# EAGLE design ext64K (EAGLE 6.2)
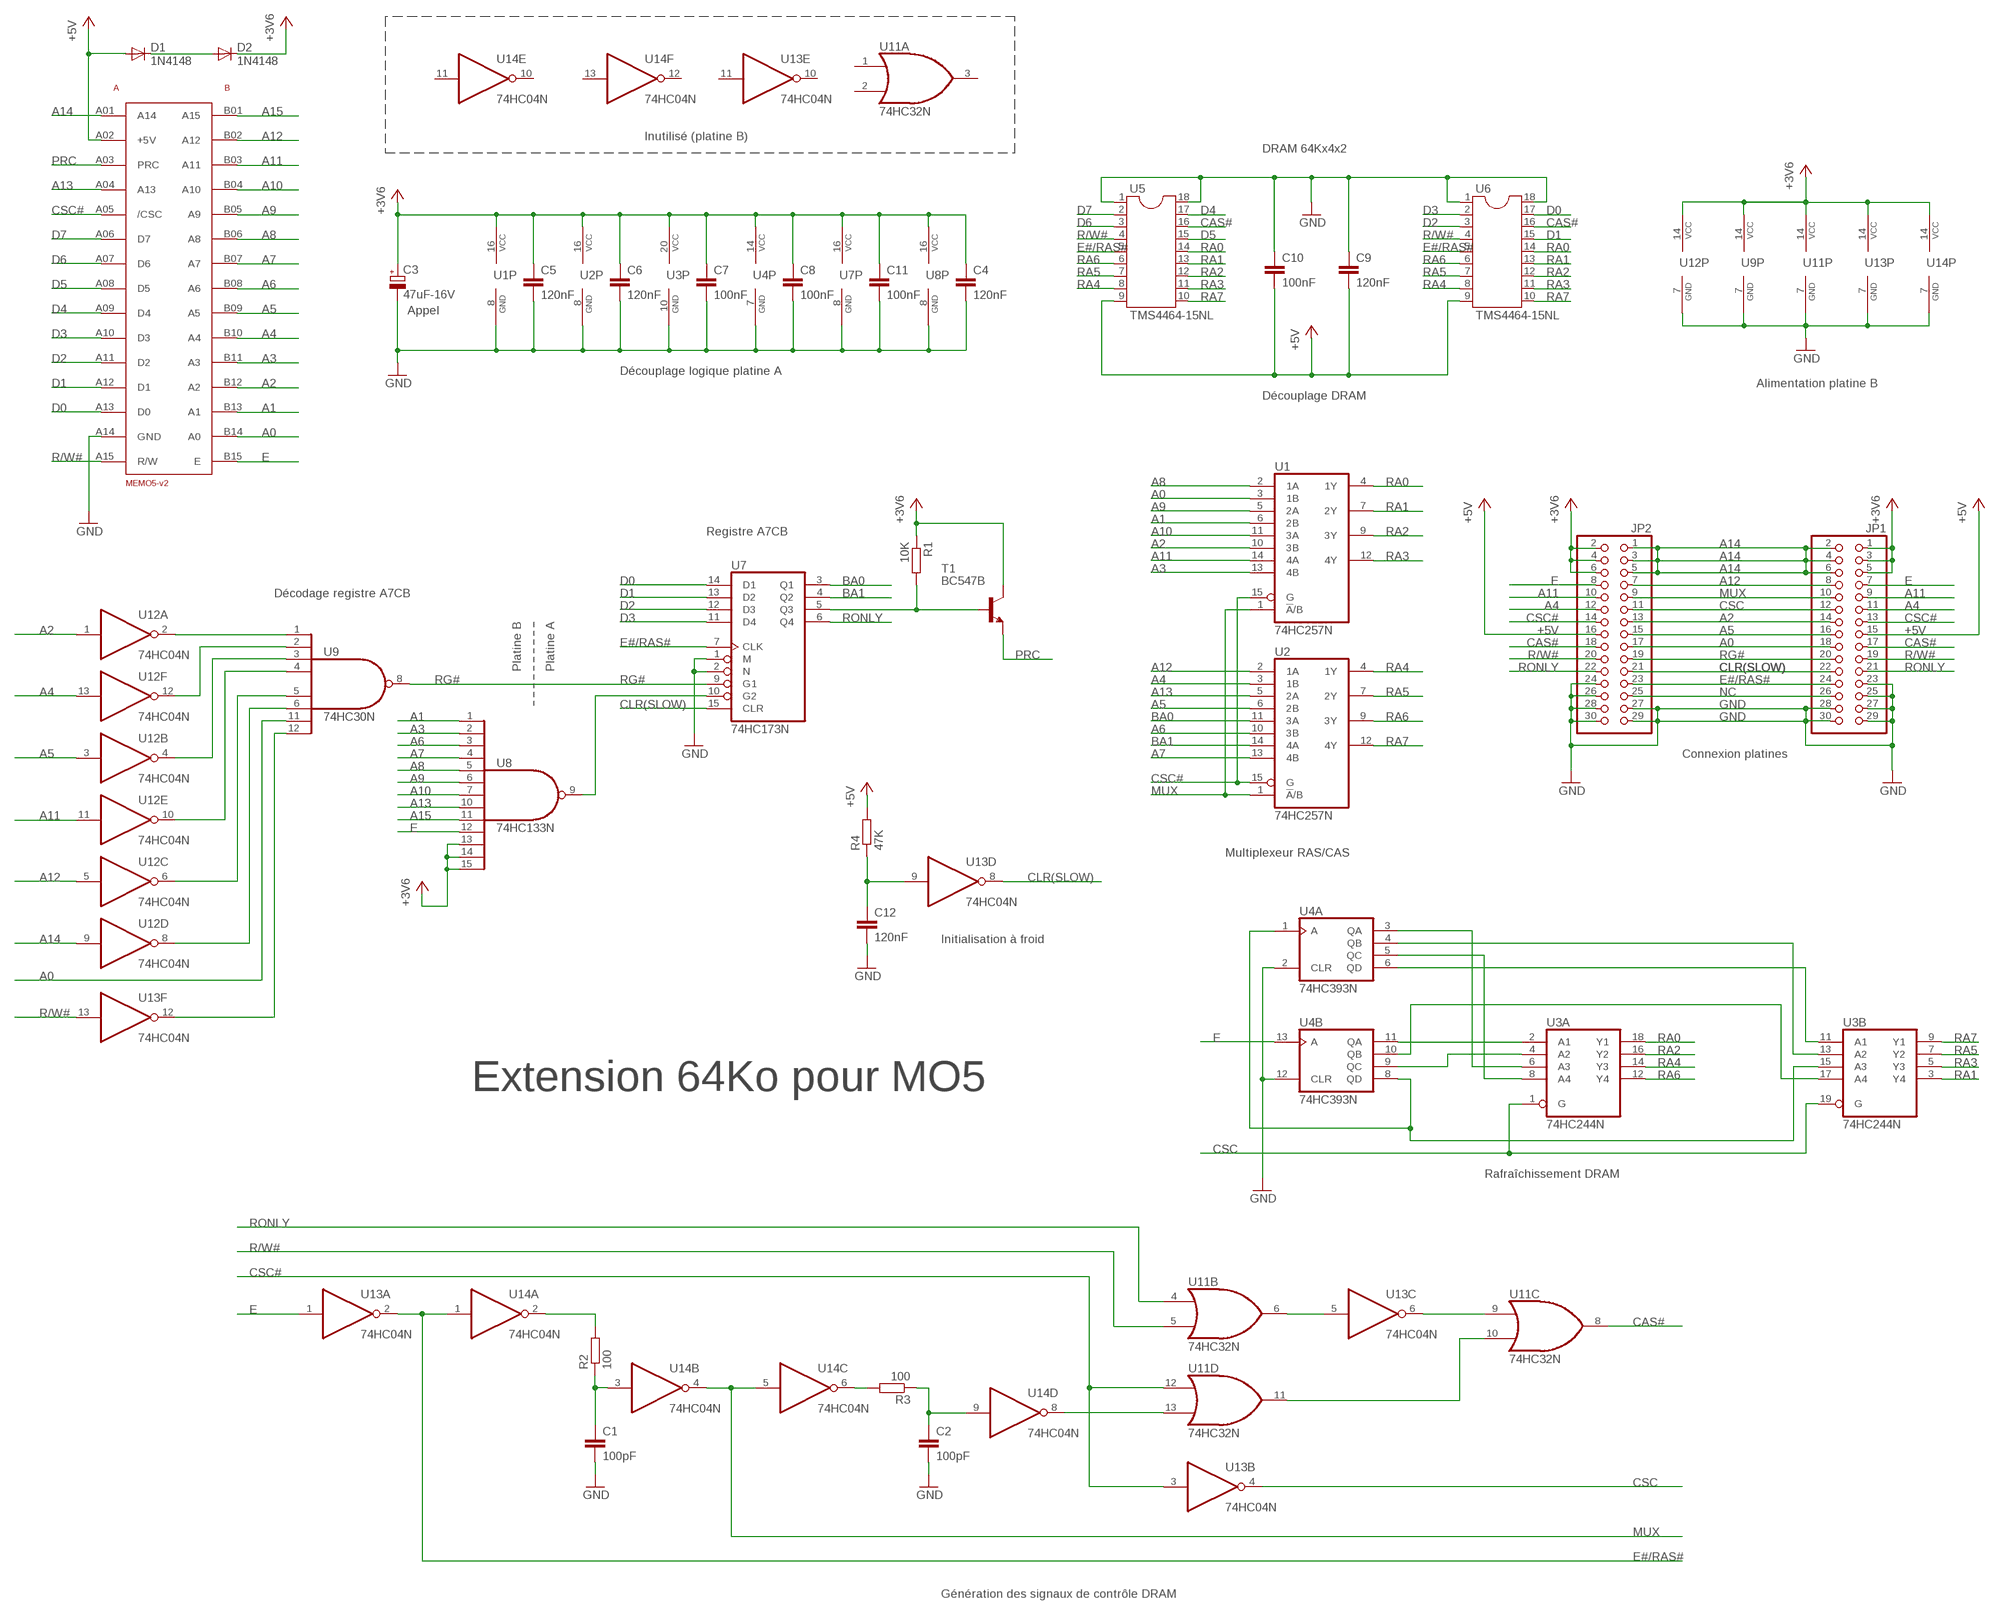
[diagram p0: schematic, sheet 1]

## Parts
BUSMO5  MEMO5-V2ST  [MEMO5]
C1  100pF  C-EU050-025X075  [C050-025X075]
C2  100pF  C-EU050-025X075  [C050-025X075]
C3  47uF-16V  CPOL-EUE5-6  [E5-6]
C4  120nF  C-EU050-024X044  [C050-024X044]
C5  120nF  C-EU050-024X044  [C050-024X044]
C6  120nF  C-EU050-024X044  [C050-024X044]
C7  100nF  C-EU050-024X044  [C050-024X044]
C8  100nF  C-EU050-024X044  [C050-024X044]
C9  120nF  C-EU050-024X044  [C050-024X044]
C10  100nF  C-EU050-024X044  [C050-024X044]
C11  100nF  C-EU050-024X044  [C050-024X044]
C12  120nF  C-EU050-024X044  [C050-024X044]
D1  1N4148  DIODE-DO15-12  [DO15-12]
D2  1N4148  DIODE-DO15-12  [DO15-12]
JP1  PINHD-2X15  [2X15]
JP2  PINHD-2X15  [2X15]
R1  10K  R-EU_0309/12  [0309/12]
R2  100  R-EU_0309/12  [0309/12]
R3  100  R-EU_0309/12  [0309/12]
R4  47K  R-EU_0309/12  [0309/12]
T1  BC547B  [TO92]
U1  74HC257N  74LS257N  [DIL16]
U2  74HC257N  74LS257N  [DIL16]
U3  74HC244N  74LS244N  [DIL20]
U4  74HC393N  74LS393N  [DIL14]
U5  TMS4464-15NL  DIL18  [DIL18]
U6  TMS4464-15NL  DIL18  [DIL18]
U7  74HC173N  74LS173N  [DIL16]
U8  74HC133N  74S133N  [DIL16]
U9  74HC30N  74ALS30N  [DIL14]
U11  74HC32N  74LS32N  [DIL14]
U12  74HC04N  74ALS04N  [DIL14]
U13  74HC04N  74AS04N  [DIL14]
U14  74HC04N  74AS04N  [DIL14]

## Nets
+3V6: C3.+ C4.1 C5.1 C6.1 C7.1 C8.1 C11.1 D2.C JP1.1 JP1.3 JP1.5 JP2.2 JP2.4 JP2.6 R1.1 T1.3(C) U1.16(VCC) U2.16(VCC) U3.20(P:VCC) U4.14(P:VCC) U7.16(VCC) U8.13(I10) U8.14(I11) U8.15(I12) U8.16(VCC) U9.14(VCC) U11.14(P:VCC) U12.14(P:VCC) U13.14(P:VCC) U14.14(P:VCC)
+5V: BUSMO5.A02(+5V) C9.2 C10.2 D1.A JP1.15 JP2.16 R4.2 U5.9 U6.9
A0: BUSMO5.B14(A0) JP1.18 JP2.17 U1.3(1B) U9.11(I6)
A1: BUSMO5.B13(A1) U1.6(2B) U8.1(I0)
A2: BUSMO5.B12(A2) JP1.14 JP2.13 U1.10(3B) U12.1(A:I)
A3: BUSMO5.B11(A3) U1.13(4B) U8.2(I1)
A4: BUSMO5.B10(A4) JP1.11 JP2.12 U2.3(1B) U12.13(F:I)
A5: BUSMO5.B09(A5) JP1.16 JP2.15 U2.6(2B) U12.3(B:I)
A6: BUSMO5.B08(A6) U2.10(3B) U8.3(I2)
A7: BUSMO5.B07(A7) U2.13(4B) U8.4(I3)
A8: BUSMO5.B06(A8) U1.2(1A) U8.5(I4)
A9: BUSMO5.B05(A9) U1.5(2A) U8.6(I5)
A10: BUSMO5.B04(A10) U1.11(3A) U8.7(I6)
A11: BUSMO5.B03(A11) JP1.9 JP2.10 U1.14(4A) U12.11(E:I)
A12: BUSMO5.B02(A12) JP1.8 JP2.7 U2.2(1A) U12.5(C:I)
A13: BUSMO5.A04(A13) U2.5(2A) U8.10(I7)
A14: BUSMO5.A01(A14) JP1.2 JP1.4 JP1.6 JP2.1 JP2.3 JP2.5 U12.9(D:I)
A15: BUSMO5.B01(A15) U8.11(I8)
A#B(SLOW): U11.13(D:I1) U14.8(D:O)
BA0: U2.11(3A) U7.3(Q1)
BA1: U2.14(4A) U7.4(Q2)
CAS#: JP1.17 JP2.18 U5.16 U6.16 U11.8(C:O)
CLR(SLOW): JP1.22 JP2.21 U7.15(CLR) U13.8(D:O)
CSC: JP1.12 JP2.11 U3.1(A:G) U3.19(B:G) U13.4(B:O)
CSC#: BUSMO5.A05(/CSC) JP1.13 JP2.14 U1.15(G) U2.15(G) U11.12(D:I0) U13.3(B:I)
D0: BUSMO5.A13(D0) U6.17 U7.14(D1)
D1: BUSMO5.A12(D1) U6.15 U7.13(D2)
D2: BUSMO5.A11(D2) U6.3 U7.12(D3)
D3: BUSMO5.A10(D3) U6.2 U7.11(D4)
D4: BUSMO5.A09(D4) U5.17
D5: BUSMO5.A08(D5) U5.15
D6: BUSMO5.A07(D6) U5.3
D7: BUSMO5.A06(D7) U5.2
E: BUSMO5.B15(E) JP1.7 JP2.8 U4.13(B:A) U8.12(I9) U13.1(A:I)
E#/RAS#: JP1.24 JP2.23 U5.5 U6.5 U7.7(CLK) U13.2(A:O) U14.1(A:I)
E(SLOW): C1.1 R2.1 U14.3(B:I)
GND: BUSMO5.A14(GND) C1.2 C2.2 C3.- C4.2 C5.2 C6.2 C7.2 C8.2 C9.1 C10.1 C11.2 C12.2 JP1.23 JP1.25 JP1.27 JP1.28 JP1.29 JP1.30 JP2.24 JP2.26 JP2.27 JP2.28 JP2.29 JP2.30 U1.8(GND) U2.8(GND) U3.10(P:GND) U4.2(A:CLR) U4.7(P:GND) U4.12(B:CLR) U5.1 U5.18 U6.1 U6.18 U7.1(M) U7.2(N) U7.8(GND) U8.8(GND) U9.7(GND) U11.7(P:GND) U12.7(P:GND) U13.7(P:GND) U14.7(P:GND)
MUX: JP1.10 JP2.9 U1.1(!A!/B) U2.1(!A!/B) U14.4(B:O) U14.5(C:I)
N$1: U9.2(I1) U12.12(F:O)
N$2: U9.3(I2) U12.4(B:O)
N$3: U9.4(I3) U12.10(E:O)
N$4: U9.5(I4) U12.6(C:O)
N$5: U9.6(I5) U12.8(D:O)
N$6: D1.C D2.A
N$7: U3.2(A:A1) U4.11(B:QA)
N$10: U3.4(A:A2) U4.9(B:QC)
N$11: U3.6(A:A3) U4.3(A:QA)
N$13: U3.8(A:A4) U4.5(A:QC)
N$19: U9.12(I7) U13.12(F:O)
N$20: C12.1 R4.1 U13.9(D:I)
N$21: U3.15(B:A3) U4.1(A:A) U4.8(B:QD)
N$22: U7.10(G2) U8.9(O)
N$23: U3.11(B:A1) U4.6(A:QD)
N$24: U3.13(B:A2) U4.4(A:QB)
N$26: R2.2 U14.2(A:O)
N$27: U3.17(B:A4) U4.10(B:QB)
N$28: R3.2 U14.6(C:O)
N$30: C2.1 R3.1 U14.9(D:I)
N$32: U11.6(B:O) U13.5(C:I)
N$33: U11.9(C:I0) U13.6(C:O)
N$34: U11.10(C:I1) U11.11(D:O)
N$38: R1.2 T1.2(B) U7.5(Q3)
NC: JP1.26 JP2.25
PRC: BUSMO5.A03(PRC) T1.1(E)
R/W#: BUSMO5.A15(R/W) JP1.19 JP2.20 U5.4 U6.4 U11.5(B:I1) U13.13(F:I)
RA0: U1.4(1Y) U3.18(A:Y1) U5.14 U6.14
RA1: U1.7(2Y) U3.3(B:Y4) U5.13 U6.13
RA2: U1.9(3Y) U3.16(A:Y2) U5.12 U6.12
RA3: U1.12(4Y) U3.5(B:Y3) U5.11 U6.11
RA4: U2.4(1Y) U3.14(A:Y3) U5.8 U6.8
RA5: U2.7(2Y) U3.7(B:Y2) U5.7 U6.7
RA6: U2.9(3Y) U3.12(A:Y4) U5.6 U6.6
RA7: U2.12(4Y) U3.9(B:Y1) U5.10 U6.10
RG#: JP1.20 JP2.19 U7.9(G1) U9.8(O)
RONLY: JP1.21 JP2.22 U7.6(Q4) U11.4(B:I0)
S$6: U9.1(I0) U12.2(A:O)
Unconnected: U11.1(A:I0) U11.2(A:I1) U11.3(A:O) U13.10(E:O) U13.11(E:I) U14.10(E:O) U14.11(E:I) U14.12(F:O) U14.13(F:I)

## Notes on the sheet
- Inutilisé (platine B)
- DRAM 64Kx4x2
- Appel
- Découplage logique platine A
- Alimentation platine B
- Découplage DRAM
- Registre A7CB
- Décodage registre A7CB
- Platine B | Platine A
- Connexion platines
- Multiplexeur RAS/CAS
- Initialisation à froid
- Extension 64Ko pour MO5
- Rafraîchissement DRAM
- Génération des signaux de contrôle DRAM

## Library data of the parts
BUSMO5 = thomson:MEMO5-V2
C1 C2 C4-C12 = rcl:C-EU: CAPACITOR, European symbol
C3 = rcl:CPOL-EU: POLARIZED CAPACITOR, European symbol
D1 D2 = diode:DIODE-: DIODE
JP1 JP2 = pinhead:PINHD-2X15: PIN HEADER
R1-R4 = rcl:R-EU_: RESISTOR, European symbol
T1 = transistor-npn:BC547*: NPN Transistor
U1 U2 = 74xx-us:74*257: Quadruple 2-to 1 line data SELECTOR/MULTIPLEXER
U3 = 74xx-us:74*244: Octal BUFFER and LINE DRIVER, 3-state
U4 = 74xx-us:74*393: Dual 4-bit decade and binary COUNTER
U5 U6 = ic-package:DIL18: Dual In Line / Socket
U7 = 74xx-us:74*173: 4-bit D type REGISTER, 3-state
U8 = 74xx-us:74*133: 13-input NAND gate
U9 = 74xx-us:74*30: 8-input NAND gate
U11 = 74xx-us:74*32: Quad 2-input OR gate
U12-U14 = 74xx-us:74*04: Hex INVERTER

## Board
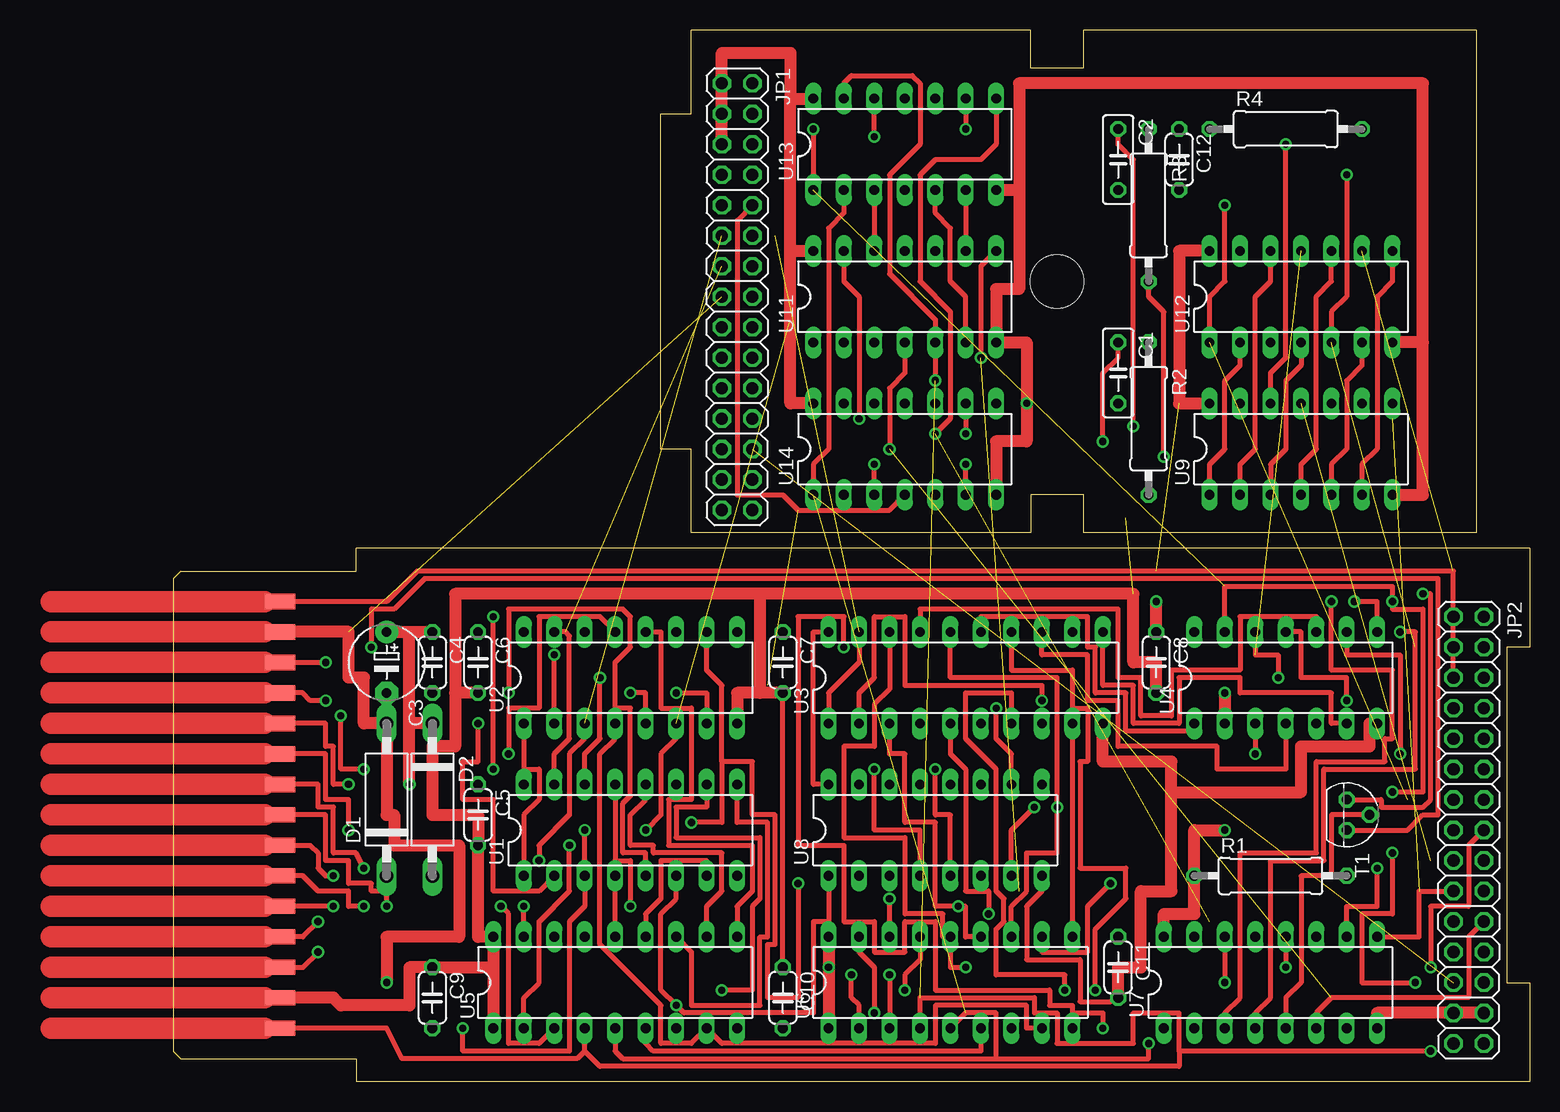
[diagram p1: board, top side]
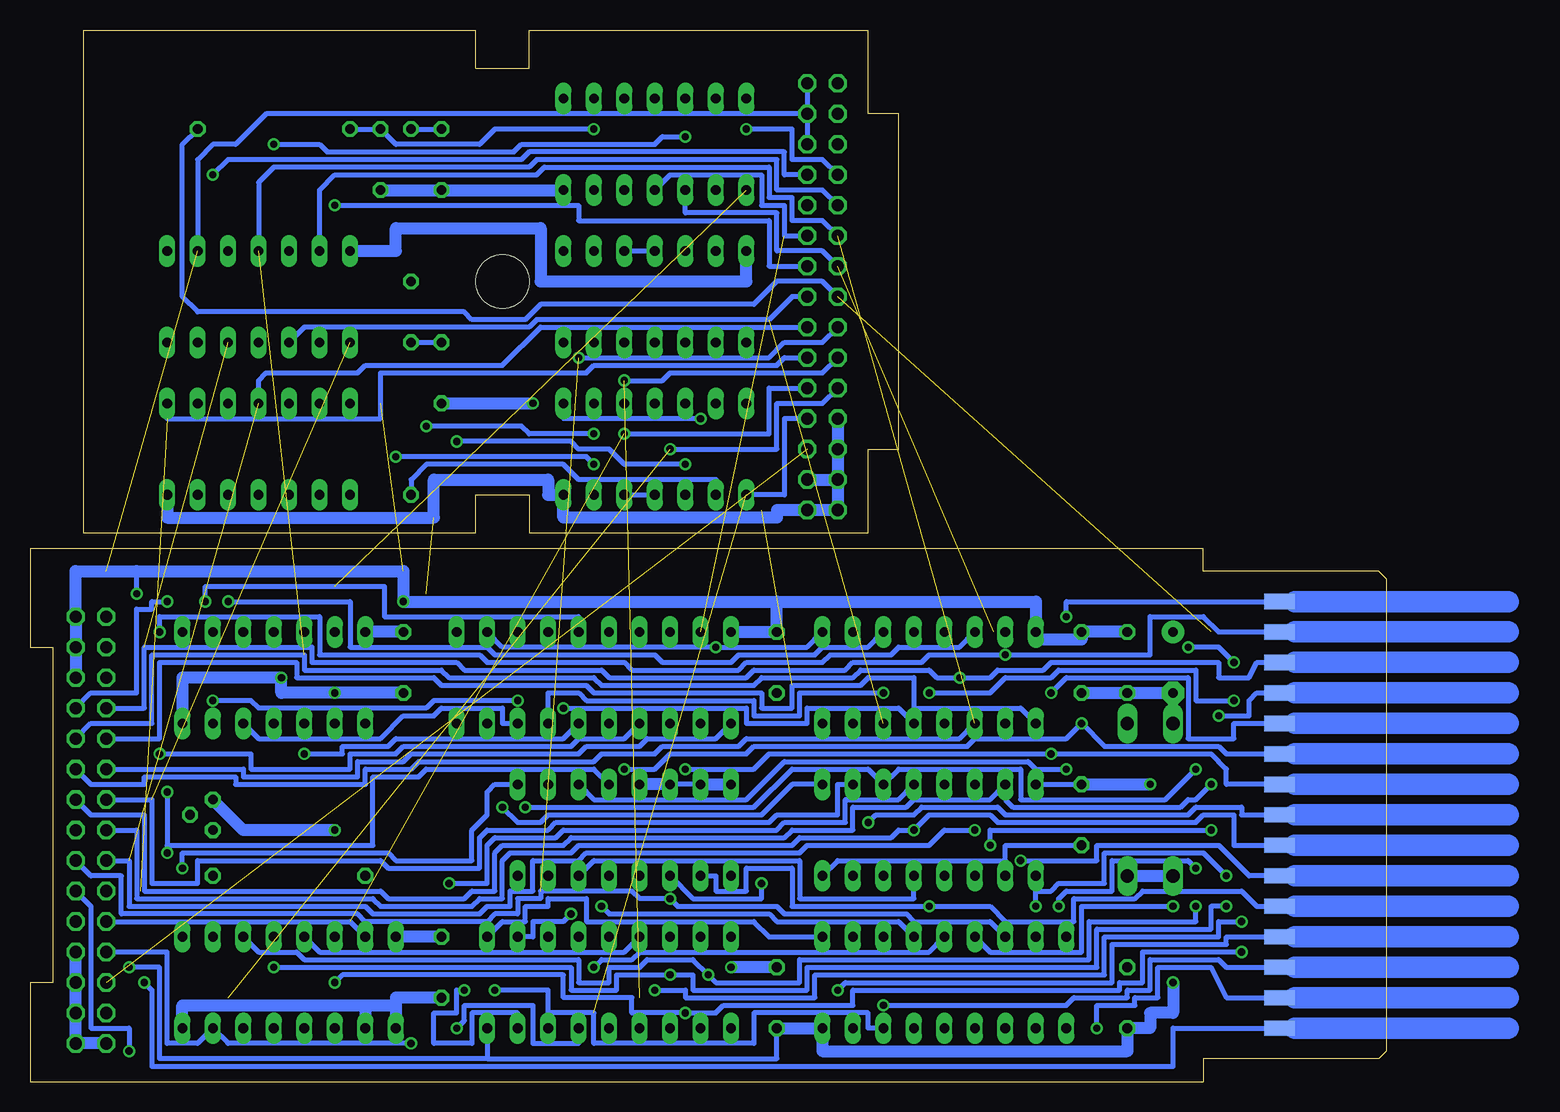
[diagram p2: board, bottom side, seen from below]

Size 113.03 x 87.63 mm. Coordinates in mm from the lower left corner, seen from the top.
Outline: 108.59,87.63 108.59,45.72 75.88,45.72 75.88,48.89 71.44,48.89 71.44,45.72 43.18,45.72 43.18,52.7 40.64,52.7 40.64,80.64 43.18,80.64 43.18,87.63 71.44,87.63 71.44,84.45 75.88,84.45 75.88,87.63 108.59,87.63
Outline: 113.03,44.45 15.24,44.45 15.24,42.54 0.63,42.54 0,41.91 0,2.54 0.63,1.9 15.24,1.9 15.24,0 113.03,0 113.03,8.25 111.12,8.25 111.12,36.2 113.03,36.2 113.03,44.45
Copper layers (1*16): Top 0.035mm / dielectric 1.5mm / Bottom 0.035mm
Design rules: minimum track width 10mil, minimum drill 24mil, track to track 8mil, track to pad 8mil, pad to pad 8mil, via to via 8mil, smd to smd 8mil, copper to edge 40mil, drill to drill 8mil, minimum pad ring 10mil, minimum via ring 8mil, stop-mask expansion 4mil, vias tented up to drill 0mil, thermal gap 10mil
Holes 4.45 mm at 73.66,66.67

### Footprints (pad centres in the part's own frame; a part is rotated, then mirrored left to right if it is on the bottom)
MEMO5 = smd 1.27 x 2.54: A01 -17.78,0; A02 -15.24,0; A03 -12.7,0; A04 -10.16,0; A05 -7.62,0; A06 -5.08,0; A07 -2.54,0; A08 0,0; A09 2.54,0; A10 5.08,0; A11 7.62,0; A12 10.16,0; A13 12.7,0; A14 15.24,0; A15 17.78,0 | smd 1.27 x 2.54 bottom: B01 -17.78,0; B02 -15.24,0; B03 -12.7,0; B04 -10.16,0; B05 -7.62,0; B06 -5.08,0; B07 -2.54,0; B08 0,0; B09 2.54,0; B10 5.08,0; B11 7.62,0; B12 10.16,0; B13 12.7,0; B14 15.24,0; B15 17.78,0
C050-025X075 = drill 0.813 octagon: 1 -2.54,0; 2 2.54,0
E5-6 = drill 0.813 pad 1.905: + -2.54,0 | drill 0.813 pad 1.905 octagon: - 2.54,0
C050-024X044 = drill 0.813 octagon: 1 -2.54,0; 2 2.54,0
DO15-12 = drill 1.118 long: A 6.35,0; C -6.35,0
2X15 = drill 1.016 octagon: 1 -17.78,-1.27; 2 -17.78,1.27; 3 -15.24,-1.27; 4 -15.24,1.27; 5 -12.7,-1.27; 6 -12.7,1.27; 7 -10.16,-1.27; 8 -10.16,1.27; 9 -7.62,-1.27; 10 -7.62,1.27; 11 -5.08,-1.27; 12 -5.08,1.27; 13 -2.54,-1.27; 14 -2.54,1.27; 15 0,-1.27; 16 0,1.27; 17 2.54,-1.27; 18 2.54,1.27; 19 5.08,-1.27; 20 5.08,1.27; 21 7.62,-1.27; 22 7.62,1.27; 23 10.16,-1.27; 24 10.16,1.27; 25 12.7,-1.27; 26 12.7,1.27; 27 15.24,-1.27; 28 15.24,1.27; 29 17.78,-1.27; 30 17.78,1.27
0309/12 = drill 0.813 octagon: 1 -6.35,0; 2 6.35,0
TO92 = drill 0.813 octagon: 1 1.27,0; 2 0,1.905; 3 -1.27,0
DIL16 = drill 0.813 long: 1 -8.89,-3.81; 2 -6.35,-3.81; 3 -3.81,-3.81; 4 -1.27,-3.81; 5 1.27,-3.81; 6 3.81,-3.81; 7 6.35,-3.81; 8 8.89,-3.81; 9 8.89,3.81; 10 6.35,3.81; 11 3.81,3.81; 12 1.27,3.81; 13 -1.27,3.81; 14 -3.81,3.81; 15 -6.35,3.81; 16 -8.89,3.81
DIL20 = drill 0.813 long: 1 -11.43,-3.81; 2 -8.89,-3.81; 3 -6.35,-3.81; 4 -3.81,-3.81; 5 -1.27,-3.81; 6 1.27,-3.81; 7 3.81,-3.81; 8 6.35,-3.81; 9 8.89,-3.81; 10 11.43,-3.81; 11 11.43,3.81; 12 8.89,3.81; 13 6.35,3.81; 14 3.81,3.81; 15 1.27,3.81; 16 -1.27,3.81; 17 -3.81,3.81; 18 -6.35,3.81; 19 -8.89,3.81; 20 -11.43,3.81
DIL14 = drill 0.813 long: 1 -7.62,-3.81; 2 -5.08,-3.81; 3 -2.54,-3.81; 4 0,-3.81; 5 2.54,-3.81; 6 5.08,-3.81; 7 7.62,-3.81; 8 7.62,3.81; 9 5.08,3.81; 10 2.54,3.81; 11 0,3.81; 12 -2.54,3.81; 13 -5.08,3.81; 14 -7.62,3.81
DIL18 = drill 0.813 long: 1 -10.16,-3.81; 2 -7.62,-3.81; 3 -5.08,-3.81; 4 -2.54,-3.81; 5 0,-3.81; 6 2.54,-3.81; 7 5.08,-3.81; 8 7.62,-3.81; 9 10.16,-3.81; 10 10.16,3.81; 11 7.62,3.81; 12 5.08,3.81; 13 2.54,3.81; 14 0,3.81; 15 -2.54,3.81; 16 -5.08,3.81; 17 -7.62,3.81; 18 -10.16,3.81

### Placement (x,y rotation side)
BUSMO5  8.89,22.23 270 top
C1  78.74,59.05 270 top
C2  78.74,76.83 270 top
C3  17.78,34.92 270 top
C4  21.59,34.92 270 top
C5  25.4,22.23 270 top
C6  25.4,34.92 270 top
C7  50.8,34.92 270 top
C8  81.92,34.92 270 top
C9  21.59,6.98 270 top
C10  50.8,6.98 270 top
C11  78.74,9.52 270 top
C12  83.82,76.83 270 top
D1  17.78,23.5 90 top
D2  21.59,23.5 270 top
JP1  46.99,65.41 270 top
JP2  107.95,20.96 270 top
R1  91.44,17.14 0 top
R2  81.28,55.24 270 top
R3  81.28,73.02 270 top
R4  92.71,79.38 0 top
T1  97.79,22.23 270 top
U1  38.1,20.96 0 top
U2  38.1,33.66 0 top
U3  66.04,33.66 0 top
U4  92.71,33.66 0 top
U5  36.83,8.25 0 top
U6  64.77,8.25 0 top
U7  91.44,8.25 0 top
U8  63.5,20.96 0 top
U9  93.98,52.7 0 top
U11  60.96,65.41 0 top
U12  93.98,65.41 0 top
U13  60.96,78.11 0 top
U14  60.96,52.7 0 top

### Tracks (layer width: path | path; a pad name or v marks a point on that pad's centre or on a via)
+3V6  (via drill 0.6)  (1 unrouted)
  Top 0.406: T1.3 100.65,23.5 100.65,22.86 104.14,22.86 104.78,23.5 104.78,40.64 v104.14,40.64 | U8.16 53.34,24.77 53.34,37.46 U3.20
  Top 1.016: U12.14 83.82,69.22 83.82,56.52 U9.14 | U14.14 51.43,56.52 51.43,69.22 | 51.43,69.22 U11.14 | 51.43,69.22 51.43,81.91 | 51.43,81.91 U13.14 | JP1.5 JP1.3 JP1.1 45.72,85.72 51.43,85.72 51.43,81.91 | C8.1 v81.92,40 | C3.+ 19.68,37.46 | 19.68,37.46 C4.1 | D2.C 19.68,29.85 | 19.68,29.85 19.68,37.46 | U7.16 82.55,13.97 85.09,13.97 R1.1 85.09,20.96 v87.63,20.96 | v19.68,24.77 19.68,29.85
  Bottom 0.406: v104.14,40.64 104.14,42.54 | U8.15 U8.14 | U1.16 C5.1
  Bottom 1.016: U12.14 82.55,69.22 82.55,71.12 70.48,71.12 70.48,66.67 53.34,66.67 U11.14 | C8.1 U4.14 | JP2.6 JP2.4 JP2.2 109.22,42.54 104.14,42.54 81.92,42.54 v81.92,40 50.8,40 | 50.8,40 29.21,40 U2.16 29.21,36.83 25.4,36.83 C6.1 C4.1 | 50.8,40 C7.1 U3.20 | v87.63,20.96 95.25,20.96 T1.3 | C11.1 U7.16 | U8.15 U8.16 | U8.14 U8.13 | C5.1 v19.68,24.77
+5V  (via drill 0.6)  (1 unrouted)
  Top 0.406: JP2.16 107.95,19.69 107.95,14.61 104.78,14.61 v104.78,9.52
  Top 1.016: BUSMO5.A02 14.61,37.46 14.61,33.66 15.88,33.66 15.88,29.85 D1.A 17.78,22.23 18.41,22.23 18.41,19.69 23.81,19.69 23.81,12.07 17.78,12.07 v17.78,8.25
  Bottom 0.406: v104.78,9.52 102.23,9.52 102.23,1.9 74.93,1.9 | U6.9 74.93,1.9 | 74.93,1.9 50.8,1.9 C10.2 | R4.2 100.33,78.11 100.33,65.41 99.06,64.14 76.84,64.14 76.2,63.5 71.76,63.5 70.48,64.77 52.7,64.77 50.8,66.67 46.99,66.67 JP1.15
  Bottom 1.016: C10.2 U5.9 46.99,2.54 21.59,2.54 C9.2 19.68,4.45 19.68,5.71 17.78,5.71 v17.78,8.25
A0  (via drill 0.6)  (1 unrouted)
  Top 0.406: v34.29,20.96 U1.3 34.29,14.61 33.02,13.34 33.02,2.54 24.13,2.54 v24.13,4.45
  Bottom 0.406: JP2.17 104.78,18.41 104.78,14.61 85.09,14.61 84.45,13.97 75.56,13.97 74.93,14.61 73.03,14.61 73.03,15.88 71.12,15.88 71.12,18.41 67.31,18.41 66.67,19.05 48.89,19.05 48.26,19.69 38.1,19.69 36.83,20.96 v34.29,20.96 | v24.13,4.45 24.13,6.35 20.96,6.35 20.96,6.98 19.05,6.98 19.05,9.52 14.61,9.52 13.34,6.98 BUSMO5.B14 | U9.11 93.98,58.42 93.34,59.05 85.73,59.05 85.09,59.69 73.66,59.69 70.48,62.86 JP1.18
A1  (via drill 0.6)
  Top 0.406: U8.1 54.61,13.34 53.34,13.34 53.34,5.71 42.54,5.71 v41.91,6.35 40.64,7.62 40.64,13.97 41.91,15.24 U1.6
  Bottom 0.406: v41.91,6.35 26.67,6.35 26.04,6.98 21.59,6.98 21.59,7.62 19.68,7.62 19.68,10.16 13.97,10.16 13.34,9.52 BUSMO5.B13
A2  (via drill 0.6)  (1 unrouted)
  Top 0.406: U1.10 44.45,22.86 41.91,22.86 41.91,20.32 48.89,20.32 48.89,15.24 48.26,14.61 48.26,7.62 v45.72,7.62 | U12.1 86.36,65.41 87.63,66.67 v87.63,73.02
  Bottom 0.406: JP2.13 102.87,23.5 102.87,16.51 99.06,16.51 99.06,18.41 83.82,18.41 83.19,17.78 75.56,17.78 75.56,20.32 74.93,20.96 69.85,20.96 69.22,21.59 51.43,21.59 50.8,22.23 45.72,22.23 45.72,24.77 U1.10 | v45.72,7.62 45.09,8.25 22.86,8.25 22.86,11.43 13.34,11.43 13.34,12.07 BUSMO5.B12 | v87.63,73.02 67.31,73.02 67.31,71.75 51.43,71.75 51.43,67.94 JP1.14
A3  (via drill 0.6)
  Top 0.406: U1.13 36.83,18.41 38.1,18.41 v38.1,14.61
  Bottom 0.406: U8.2 55.88,17.14 55.88,15.88 53.34,15.88 53.34,17.78 49.53,17.78 49.53,14.61 v38.1,14.61 33.02,14.61 31.75,13.34 26.04,13.34 26.04,15.24 20.96,15.24 20.32,15.88 12.07,15.88 10.79,14.61 BUSMO5.B11
A4  (via drill 0.6)  (1 unrouted)
  Top 0.406: U2.3 34.29,28.57 33.02,27.3 33.02,22.23 30.48,19.69 v30.48,18.41
  Bottom 0.406: JP2.12 107.95,24.77 103.51,24.77 103.51,25.4 95.89,25.4 95.89,24.77 85.09,24.77 85.09,26.04 81.28,26.04 80.65,26.67 66.04,26.67 65.41,27.3 60.96,27.3 60.32,27.94 53.97,27.94 53.34,28.57 35.56,28.57 U2.3 | v30.48,18.41 24.13,18.41 24.13,19.69 13.97,19.69 11.43,17.14 BUSMO5.B10 | U12.13 88.9,74.3 87.63,75.56 70.8,75.56 70.17,76.2 51.43,76.2 51.43,73.66 49.53,73.66 49.53,71.75 46.99,71.75 JP1.11
A5  (via drill 0.6)  (1 unrouted)
  Top 0.406: U2.6 41.91,28.57 40.64,27.3 40.64,22.23 v39.37,20.96
  Bottom 0.406: JP2.15 104.14,20.96 104.14,15.24 84.45,15.24 83.82,14.61 76.2,14.61 75.56,15.24 73.66,15.24 73.66,18.41 73.03,19.05 67.95,19.05 67.31,19.69 49.53,19.69 48.89,20.32 41.27,20.32 40.64,20.96 v39.37,20.96 38.1,22.23 33.02,22.23 32.38,21.59 15.88,21.59 15.24,22.23 12.7,22.23 12.7,19.69 BUSMO5.B09 | JP1.16 49.53,65.41 51.43,63.5 70.8,63.5 71.44,62.86 90.17,62.86 U12.3
A6  (via drill 0.6)
  Top 0.406: v52.07,16.51 52.07,6.98 49.53,6.98 49.53,11.43 50.16,11.43 50.16,22.23 48.26,22.23 48.26,26.67 45.72,26.67 | 45.72,26.67 45.72,33.02 44.45,34.29 U2.10 | 45.72,26.67 45.72,21.59 v43.18,21.59
  Bottom 0.406: U8.3 57.78,15.24 52.07,15.24 v52.07,16.51 | v43.18,21.59 42.54,22.23 39.37,22.23 38.73,22.86 32.38,22.86 31.75,22.23 16.51,22.23 15.88,22.86 12.07,22.86 12.07,22.23 BUSMO5.B08
A7  (via drill 0.6)
  Top 0.406: U8.4 62.23,20.96 58.42,20.96 v58.42,26.04 | U2.13 35.56,38.73 30.48,38.73 30.48,31.12 27.94,31.12 v27.94,27.3
  Bottom 0.406: v58.42,26.04 52.7,26.04 51.43,27.3 v27.94,27.3 14.61,27.3 13.34,26.04 13.34,24.77 BUSMO5.B07
A8  (via drill 0.6)
  Top 0.406: U8.5 64.77,22.23 63.5,22.23 v63.5,26.04 | U1.2 30.48,15.88 26.67,15.88 26.67,23.5 24.13,23.5 24.13,26.67 25.4,26.67 v25.4,29.85
  Bottom 0.406: v63.5,26.04 60.96,26.04 59.69,27.3 53.34,27.3 52.7,27.94 34.92,27.94 34.29,28.57 26.67,28.57 v25.4,29.85 23.5,27.94 13.97,27.94 13.34,27.3 BUSMO5.B06
A9  (via drill 0.6)
  Top 0.406: U1.5 39.37,19.05 37.46,19.05 37.46,23.18 38.1,23.81 38.1,31.12 36.83,31.12 36.83,34.92 38.1,36.2 38.1,38.73 37.46,39.37 27.94,39.37 v27.94,32.38
  Bottom 0.406: U8.6 66.04,18.41 48.89,18.41 48.89,15.24 39.37,15.24 U1.5 | v27.94,32.38 26.67,33.66 16.51,33.66 16.51,28.57 12.7,28.57 12.7,29.85 BUSMO5.B05
A10  (via drill 0.6)
  Top 0.406: U8.7 69.85,20.96 v71.76,22.86 | v15.88,26.04 13.97,26.04 v13.97,30.48
  Bottom 0.406: v71.76,22.86 52.7,22.86 49.53,26.04 43.18,26.04 U1.11 40.64,26.04 30.48,26.04 30.48,23.5 18.41,23.5 v15.88,26.04 | v13.97,30.48 11.43,30.48 11.43,31.75 10.79,32.38 BUSMO5.B04
A11  (via drill 0.6)  (1 unrouted)
  Top 0.406: U1.14 34.29,27.3 35.56,28.57 v35.56,33.66
  Bottom 0.406: JP2.10 107.95,29.85 102.87,29.85 102.87,35.56 90.17,35.56 90.17,34.29 78.74,34.29 78.11,33.66 66.04,33.66 65.41,33.02 52.7,33.02 52.07,33.66 44.45,33.66 43.81,34.29 38.1,34.29 37.46,33.66 v35.56,33.66 33.02,33.66 32.38,34.29 28.57,34.29 27.94,34.92 13.97,34.92 13.97,33.66 11.43,33.66 10.79,34.92 BUSMO5.B03 | JP1.9 46.99,74.3 50.8,74.3 50.8,76.83 70.8,76.83 71.44,76.2 92.71,76.2 93.98,74.93 U12.11
A12  (via drill 0.6)  (1 unrouted)
  Top 0.406: U2.2 v31.75,35.56 | v97.79,75.56 97.79,65.41 96.52,64.14 U12.5
  Bottom 0.406: JP2.7 103.51,31.12 103.51,36.2 89.54,36.2 89.54,34.92 77.47,34.92 76.84,34.29 65.41,34.29 64.77,33.66 53.34,33.66 52.7,34.29 45.09,34.29 44.45,34.92 38.73,34.92 38.1,35.56 v31.75,35.56 19.68,35.56 19.68,38.73 15.24,38.73 13.97,37.46 BUSMO5.B02 | JP1.8 50.16,75.56 50.16,77.47 71.44,77.47 72.07,76.83 96.52,76.83 v97.79,75.56
A13  (via drill 0.6)
  Top 0.406: U8.10 69.85,27.3 68.58,28.57 v68.58,31.12 | U2.5 39.37,32.38 v38.1,32.38 | v12.7,31.75 11.43,31.75 10.79,32.38 BUSMO5.A04
  Bottom 0.406: v68.58,31.12 53.34,31.12 53.34,29.85 48.26,29.85 48.26,31.12 40.64,31.12 U2.5 | v38.1,32.38 33.02,32.38 31.75,33.66 27.94,33.66 27.3,34.29 15.88,34.29 15.88,31.75 v12.7,31.75
A14  (1 unrouted)
  Top 0.406: JP2.5 JP2.3 JP2.1 106.68,42.54 20.32,42.54 17.78,40 BUSMO5.A01
  Bottom 0.406: JP1.2 JP1.4 | JP1.4 JP1.6 | JP1.4 93.34,80.64 95.89,78.11 97.79,78.11 99.06,76.83 U12.9
A15  (via drill 0.6)
  Top 0.406: v26.67,26.04 v26.67,38.73
  Bottom 0.406: U8.11 66.04,23.5 53.34,23.5 50.16,26.67 29.85,26.67 29.21,26.04 v26.67,26.04 | v26.67,38.73 26.67,40 BUSMO5.B01
A#B(SLOW)  (via drill 0.6)
  Top 0.406: U11.13 55.88,66.67 57.15,65.41 v57.15,55.24
  Bottom 0.406: v57.15,55.24 68.58,55.24 U14.8
BA0  (via drill 0.6)
  Top 0.406: U7.3 87.63,5.71 88.9,6.98 88.9,19.05 95.25,19.05 95.25,26.67 100.97,26.67 100.97,28.57 101.6,28.57 101.6,34.29 96.52,34.29 v96.52,40
  Bottom 0.406: v96.52,40 86.36,40 86.36,36.2 74.93,36.2 74.3,35.56 60.96,35.56 60.32,34.92 54.61,34.92 53.97,35.56 47.62,35.56 46.99,36.2 43.18,36.2 U2.11
BA1  (via drill 0.6)
  Top 0.406: U7.4 90.17,5.71 91.44,6.98 91.44,18.41 95.89,18.41 95.89,26.04 103.51,26.04 103.51,37.46 v102.23,37.46
  Bottom 0.406: v102.23,37.46 102.23,38.73 88.9,38.73 88.9,35.56 75.56,35.56 74.93,34.92 63.5,34.92 62.86,34.29 53.97,34.29 53.34,34.92 46.99,34.92 46.35,35.56 41.27,35.56 40.64,36.2 35.56,36.2 U2.14
CAS#  (via drill 0.6)  (1 unrouted)
  Top 0.406: U6.16 v59.69,15.24 | U11.8 67.31,67.94 v67.31,60.32
  Bottom 0.406: JP2.18 107.95,17.14 105.41,17.14 105.41,13.97 85.73,13.97 85.09,13.34 74.93,13.34 74.3,13.97 72.39,13.97 72.39,15.24 70.48,15.24 70.48,15.88 62.86,15.88 62.23,15.24 v59.69,15.24 59.05,14.61 50.8,14.61 50.16,13.97 40,13.97 39.37,13.34 33.02,13.34 U5.16 | v67.31,60.32 51.43,60.32 50.16,61.59 46.99,61.59 JP1.17
CLR(SLOW)  (via drill 0.6)  (1 unrouted)
  Top 0.406: U13.8 68.58,78.11 67.31,76.83 63.5,76.83 62.23,75.56 62.23,66.67 64.77,64.14 64.77,55.24 v63.5,53.97
  Bottom 0.406: JP2.21 86.36,13.34 U7.15 | v63.5,53.97 51.43,53.97 51.43,57.78 JP1.22
CSC  (1 unrouted)
  Top 0.406: U3.19 57.15,34.92 54.61,32.38 U3.1
  Bottom 0.406: JP2.11 95.25,26.04 95.25,25.4 85.73,25.4 85.73,26.67 81.92,26.67 81.28,27.3 67.31,27.3 66.67,27.94 62.23,27.94 61.59,28.57 55.88,28.57 U3.1 | U13.4 59.69,75.56 52.07,75.56 52.07,73.02 50.16,73.02 50.16,70.48 JP1.12
CSC#  (via drill 0.6)  (1 unrouted)
  Top 0.406: U1.15 31.75,27.3 33.02,28.57 33.02,37.15 32.7,37.46 U2.15 | v14.61,24.77 13.34,24.77 13.34,27.94 12.7,27.94 12.7,29.85 BUSMO5.A05 | U13.3 U11.12
  Bottom 0.406: JP2.14 107.95,22.23 103.51,22.23 103.51,15.88 83.82,15.88 83.19,15.24 76.84,15.24 76.2,15.88 74.3,15.88 74.3,19.05 73.66,19.69 68.58,19.69 67.95,20.32 50.16,20.32 49.53,20.96 44.45,20.96 44.45,22.86 40,22.86 39.37,23.5 33.02,23.5 U1.15 31.75,23.5 31.12,22.86 17.14,22.86 16.51,23.5 15.88,23.5 v14.61,24.77 | JP1.13 46.99,69.22 50.8,69.22 50.8,72.39 58.42,72.39 U13.3
D0  (via drill 0.6)
  Top 0.406: U6.17 57.15,10.79 58.42,9.52 v58.42,5.71 | U7.14 v87.63,8.25 | BUSMO5.A13 10.79,9.52 v12.07,10.79
  Bottom 0.406: v87.63,8.25 87,8.89 68.58,8.89 68.58,6.98 62.86,6.98 62.86,5.71 v58.42,5.71 55.88,5.71 55.24,6.35 44.45,6.35 44.45,7.62 22.23,7.62 22.23,8.25 20.32,8.25 20.32,10.79 v12.07,10.79
D1  (via drill 0.6)
  Top 0.406: U6.15 62.23,10.16 60.96,8.89 v60.96,7.62 | v12.07,13.34 10.79,12.07 BUSMO5.A12
  Bottom 0.406: U7.13 88.9,10.79 63.5,10.79 U6.15 | v60.96,7.62 58.42,7.62 58.42,6.98 47.62,6.98 47.62,8.89 23.5,8.89 23.5,12.07 13.97,12.07 13.97,13.34 v12.07,13.34
D2  (via drill 0.6)
  Top 0.406: U7.12 v92.71,9.52 | v59.69,8.89 U6.3 | v13.34,14.61 BUSMO5.A11
  Bottom 0.406: v92.71,9.52 67.95,9.52 67.95,7.62 64.14,7.62 64.14,8.89 v59.69,8.89 57.78,8.89 57.78,7.62 48.26,7.62 48.26,9.52 24.13,9.52 24.13,12.7 14.61,12.7 14.61,14.61 v13.34,14.61
D3  (via drill 0.6)
  Top 0.406: U6.2 57.15,6.35 56.52,6.98 v56.52,8.89 | v15.88,14.61 14.61,14.61 14.61,15.88 12.07,15.88 10.79,17.14 BUSMO5.A10
  Bottom 0.406: U7.11 93.98,10.79 90.81,10.79 90.17,10.16 67.31,10.16 67.31,8.25 64.77,8.25 64.77,9.52 62.23,9.52 61.59,10.16 57.78,10.16 v56.52,8.89 55.88,8.25 48.89,8.25 48.89,10.16 24.77,10.16 24.77,13.34 15.88,13.34 v15.88,14.61
D4  (via drill 0.6)
  Top 0.406: U5.17 v29.21,14.61 | BUSMO5.A09 11.43,19.69 12.07,19.05 12.07,17.78 12.7,17.14 v13.34,17.14
  Bottom 0.406: v29.21,14.61 29.21,15.88 27.94,15.88 27.3,16.51 23.5,16.51 23.5,19.05 15.24,19.05 v13.34,17.14
D5  (via drill 0.6)
  Top 0.406: v17.78,14.61 17.78,15.88 16.51,15.88 16.51,16.51 14.61,16.51 14.61,18.41 12.7,18.41 12.7,22.23 BUSMO5.A08
  Bottom 0.406: U5.15 33.02,10.79 25.4,10.79 25.4,14.61 v17.78,14.61
D6  (via drill 0.6)
  Top 0.406: U5.3 30.48,3.17 27.94,3.17 27.94,13.97 v27.3,14.61 | v15.88,17.78 15.24,19.05 13.34,19.05 13.34,22.86 12.07,22.86 12.07,24.77 BUSMO5.A07
  Bottom 0.406: v27.3,14.61 27.3,15.24 26.67,15.88 22.86,15.88 22.86,18.41 16.51,18.41 v15.88,17.78
D7  (via drill 0.6)
  Top 0.406: U5.2 29.21,6.98 30.48,8.25 30.48,13.34 33.02,15.88 v33.02,19.69 | v14.61,20.96 14.61,23.5 12.7,23.5 12.7,27.3 BUSMO5.A06
  Bottom 0.406: v33.02,19.69 33.02,20.96 v14.61,20.96
E  (via drill 0.6)  (1 unrouted)
  Top 0.406: U4.13 87.63,41.27 101.6,41.27 v101.6,40 101.6,39.37 104.14,39.37 104.14,24.13 v101.6,24.13 | v101.6,19.05 101.6,13.97 99.06,13.97 99.06,8.25 v103.51,8.25 | v53.34,79.38 U13.1
  Bottom 0.406: v101.6,24.13 101.6,19.69 | 101.6,19.69 v101.6,19.05 | v103.51,8.25 102.87,7.62 102.87,1.27 17.78,1.27 17.78,4.45 BUSMO5.B15 | JP2.8 107.95,32.38 104.14,32.38 104.14,39.37 102.87,39.37 102.87,40 v101.6,40 | 101.6,19.69 84.45,19.69 84.45,25.4 80.65,25.4 80.01,26.04 66.04,26.04 U8.12 | JP1.7 46.99,76.83 49.53,76.83 49.53,79.38 v53.34,79.38
E#/RAS#  (via drill 0.6)  (1 unrouted)
  Top 0.406: U5.5 36.83,2.54 37.46,1.9 68.58,1.9 | v81.28,3.17 81.28,1.9 68.58,1.9 | 68.58,1.9 68.58,5.71 66.04,5.71 U6.5 | U13.2 55.88,72.39 54.61,71.12 54.61,52.7 53.34,51.43 U14.1
  Bottom 0.406: v81.28,3.17 96.52,3.17 U7.7 99.06,3.17 101.6,3.17 101.6,10.79 JP2.23 | JP1.24 50.16,55.24 50.16,48.89 U14.1
E(SLOW)  (via drill 0.6)
  Top 0.406: U14.3 v58.42,51.43 | v77.47,53.34 77.47,59.05 78.74,60.32 C1.1
  Bottom 0.406: R2.1 C1.1 | v58.42,51.43 63.5,51.43 64.77,52.7 67.31,52.7 67.95,53.34 v77.47,53.34
GND  (via drill 0.6)  (1 unrouted)
  Top 0.406: C10.1 C7.2 | U8.8 72.39,15.88 71.12,14.61 71.12,10.16 75.56,10.16 75.56,6.67 78.11,6.67 C11.2 | U4.12 90.17,35.56 92.08,35.56 v92.08,33.66
  Top 1.016: U9.7 104.14,48.89 104.14,61.59 | 104.14,61.59 U12.7 | 104.14,61.59 104.14,83.19 70.48,83.19 70.48,74.3 | 70.48,74.3 U13.7 | 70.48,74.3 70.48,66.04 68.58,66.04 U11.7 71.12,61.59 v71.12,56.52 71.12,53.34 68.58,53.34 U14.7 | JP2.28 JP2.27 100.33,5.71 U7.8 | C11.2 78.74,9.52 80.65,9.52 80.65,15.88 83.19,15.88 83.19,24.13 | 83.19,24.13 93.98,24.13 93.98,27.94 99.7,27.94 99.7,29.85 U4.7 | 83.19,24.13 83.19,26.67 77.47,26.67 U3.10 | C7.2 48.89,32.38 | 48.89,32.38 46.99,32.38 U2.8 | U6.18 v54.61,9.52 U6.1 | C8.2 81.92,34.92 80.01,34.92 80.01,40.64 48.89,40.64 | 48.89,40.64 48.89,32.38 | 48.89,40.64 23.5,40.64 23.5,32.38 | v87.63,32.38 U4.2 | C6.2 23.5,32.38 | 26.67,9.52 U5.18 25.4,12.07 C5.2 25.4,22.23 21.59,22.23 21.59,27.94 23.5,27.94 23.5,32.38 | 26.67,9.52 U5.1 | 26.67,9.52 C9.1 19.68,9.52 19.68,6.35 13.97,6.35 13.34,6.98 BUSMO5.A14
  Bottom 0.406: U1.8 45.72,18.41 31.75,18.41 31.75,19.69 C5.2
  Bottom 1.016: U9.7 101.6,46.99 79.38,46.99 79.38,50.16 69.85,50.16 69.85,48.89 U14.7 68.58,46.99 50.8,46.99 50.8,47.62 JP1.30 JP1.29 JP1.27 | JP1.23 JP1.25 JP1.27 | JP1.28 JP1.27 | C12.2 C2.2 U13.7 | C1.2 v71.12,56.52 | JP2.29 JP2.30 JP2.28 JP2.26 JP2.24 | U7.8 100.33,6.35 85.09,6.35 | 85.09,6.35 U7.2 | 85.09,6.35 82.55,6.35 | 82.55,6.35 U7.1 | C11.2 82.55,6.98 82.55,6.35 | C10.1 v54.61,9.52 | C8.2 v87.63,32.38 92.08,32.38 v92.08,33.66 100.33,33.66 U4.7 | C6.2 C4.2 C3.-
MUX  (1 unrouted)
  Top 0.406: U2.1 29.21,26.04 30.48,26.04 30.48,23.5 29.21,22.23 U1.1 | JP1.10 46.99,71.75 46.99,48.89 50.8,48.89 52.07,47.62 59.69,47.62 U14.4
  Bottom 0.406: JP2.9 102.23,28.57 102.23,34.92 90.81,34.92 90.81,33.66 79.38,33.66 78.74,33.02 66.67,33.02 66.04,32.38 52.07,32.38 52.07,31.12 49.53,31.12 49.53,33.02 43.81,33.02 43.18,33.66 39.37,33.66 39.37,31.12 30.48,31.12 U2.1 | U14.5 U14.4
N$1
  Top 0.406: U9.2 88.9,51.43 90.17,52.7 90.17,65.41 91.44,66.67 U12.12
N$2
  Top 0.406: U12.4 93.98,59.69 92.71,58.42 92.71,52.7 91.44,51.43 U9.3
N$3
  Top 0.406: U9.4 93.98,51.43 95.25,52.7 95.25,65.41 96.52,66.67 U12.10
N$4
  Top 0.406: U12.6 99.06,59.69 97.79,58.42 97.79,52.7 96.52,51.43 U9.5
N$5
  Top 0.406: U12.8 101.6,66.67 100.33,65.41 100.33,52.7 99.06,51.43 U9.6
N$6
  Bottom 1.016: D2.A D1.C
N$7  (via drill 0.6)
  Top 0.406: U3.2 57.15,32.38 58.42,33.66 58.42,38.73 60.96,38.73 60.96,33.02 72.39,33.02 v72.39,31.75 | v97.79,31.75 97.79,33.66 93.98,33.66 93.98,37.46 U4.11
  Bottom 0.406: v72.39,31.75 79.38,31.75 80.01,31.12 93.98,31.12 94.62,31.75 v97.79,31.75
N$10  (via drill 0.6)
  Top 0.406: U4.9 97.79,35.56 102.23,35.56 v102.23,27.3
  Bottom 0.406: v102.23,27.3 94.62,27.3 94.62,26.04 86.36,26.04 86.36,27.3 82.55,27.3 81.92,27.94 67.95,27.94 67.31,28.57 63.5,28.57 U3.4
N$11  (via drill 0.6)
  Top 0.406: U4.3 v90.17,27.3
  Bottom 0.406: v90.17,27.3 87,27.3 87,27.94 83.19,27.94 82.55,28.57 68.58,28.57 U3.6
N$13
  Bottom 0.406: U4.5 93.98,28.57 83.82,28.57 81.92,30.48 79.38,30.48 78.74,31.12 73.66,31.12 73.66,29.85 U3.8
N$19  (via drill 0.6)
  Top 0.406: U9.12 91.44,59.05 92.71,60.32 v92.71,78.11 | v58.42,78.74 U13.12
  Bottom 0.406: v92.71,78.11 88.9,78.11 88.27,77.47 72.71,77.47 72.07,78.11 60.96,78.11 60.32,78.74 v58.42,78.74
N$20  (via drill 0.6)
  Top 0.406: U13.9 v66.04,79.38
  Bottom 0.406: R4.1 C12.1 82.55,78.11 75.56,78.11 74.3,79.38 v66.04,79.38
N$21  (via drill 0.6)
  Top 0.406: U4.8 100.33,40 v98.43,40 | U4.1 84.45,29.21 79.38,29.21 79.38,32.38 76.84,32.38 76.84,36.2 76.2,36.2 76.2,38.73 67.31,38.73 U3.15
  Bottom 0.406: v98.43,40 98.43,41.27 83.5,41.27 83.5,38.73 67.31,38.73 U3.15
N$22  (via drill 0.6)
  Top 0.406: U7.10 97.79,14.61 100.33,14.61 v100.33,17.78
  Bottom 0.406: v100.33,17.78 100.33,19.05 83.19,19.05 82.55,18.41 76.2,18.41 76.2,20.96 74.93,22.23 74.93,24.13 74.3,24.77 U8.9
N$23
  Top 0.406: U4.6 96.52,29.85 96.52,32.38 88.9,32.38 88.9,33.66 83.82,33.66 83.82,29.85 80.01,29.85 80.01,33.02 77.47,33.02 U3.11
N$24
  Top 0.406: U4.4 92.71,26.04 87,26.04 87,27.94 78.74,27.94 78.74,31.75 76.2,31.75 76.2,35.56 72.39,35.56 U3.13
N$26
  Bottom 0.406: U14.2 55.88,50.16 67.31,50.16 68.58,51.43 80.01,51.43 81.28,50.16 R2.2
N$27
  Top 0.406: U4.10 95.25,38.73 88.9,38.73 88.9,34.29 83.19,34.29 83.19,30.48 80.65,30.48 80.65,33.66 78.74,33.66 78.74,39.37 62.23,39.37 U3.17
N$28  (via drill 0.6)
  Top 0.406: U14.6 v66.04,51.43 | v82.55,52.07 82.55,64.14 81.28,65.41 R3.2
  Bottom 0.406: v66.04,51.43 66.67,52.07 v82.55,52.07
N$30  (via drill 0.6)
  Top 0.406: U14.9 v66.04,53.97 | v80.01,54.61 80.01,76.83 78.74,78.11 C2.1
  Bottom 0.406: R3.1 C2.1 | v66.04,53.97 71.44,53.97 72.07,54.61 v80.01,54.61
N$32
  Top 0.406: U11.6 66.04,65.41 64.77,66.67 64.77,71.12 63.5,72.39 U13.5
N$33
  Top 0.406: U13.6 U11.9
N$34
  Bottom 0.406: U11.10 U11.11
N$38
  Top 0.406: T1.2 96.52,22.23 96.52,17.14 | 96.52,17.14 R1.2 | 96.52,17.14 93.98,17.14 93.98,8.25 92.71,6.98 U7.5
NC  (1 unrouted)
PRC  (via drill 0.6)
  Top 0.406: T1.1 102.87,20.96 104.14,22.23 105.41,22.23 105.41,41.91 20.96,41.91 18.41,39.37 16.51,39.37 v16.51,36.2 | BUSMO5.A03 v12.7,34.92
  Bottom 0.406: v12.7,34.92 13.97,36.2 v16.51,36.2
R/W#  (via drill 0.6)  (1 unrouted)
  Top 0.406: v104.78,2.54 83.82,2.54 | 83.82,2.54 83.82,5.71 80.01,5.71 80.01,3.17 73.66,3.17 73.66,5.71 71.76,5.71 71.76,6.98 62.23,6.98 U6.4 | 83.82,2.54 83.82,1.27 35.56,1.27 34.29,2.54 | 34.29,2.54 U5.4 | 34.29,2.54 33.66,1.9 19.05,1.9 17.78,4.45 BUSMO5.A15 | U13.13 55.88,83.19 56.52,83.82 61.59,83.82 62.23,83.19 62.23,78.11 59.69,75.56 59.69,67.31 63.5,63.5 U11.5 v63.5,58.42
  Bottom 0.406: JP2.20 107.95,14.61 107.95,4.45 104.78,4.45 v104.78,2.54 | v63.5,58.42 60.32,58.42 59.69,59.05 46.99,59.05 JP1.19
RA0  (via drill 0.6)
  Top 0.406: U5.14 U1.4 | v66.04,9.52 64.77,9.52 U6.14 64.14,12.07 64.14,13.97 60.96,13.97 60.96,20.32 55.88,20.32 55.88,27.94 58.42,27.94 58.42,31.43 59.69,32.7 U3.18
  Bottom 0.406: v66.04,9.52 65.41,10.16 62.86,10.16 62.23,10.79 38.1,10.79 U5.14
RA1  (via drill 0.6)
  Top 0.406: U1.7 44.45,18.41 40.64,18.41 40.64,15.24 39.37,13.97 U5.13 | U6.13 66.04,12.07 66.04,14.61 v65.41,14.61 63.5,14.61 63.5,21.59 60.96,21.59 60.96,27.3 59.69,27.3 U3.3
  Bottom 0.406: v65.41,14.61 64.77,13.97 51.43,13.97 50.8,13.34 40.64,13.34 U5.13
RA2  (via drill 0.6)
  Top 0.406: U6.12 69.85,14.61 71.12,15.88 71.12,19.05 73.66,19.05 v73.66,22.86 73.66,33.66 64.77,33.66 U3.16 | U5.12 43.18,10.79 43.18,6.35 48.89,6.35 48.89,12.07 49.53,12.07 49.53,21.59 46.99,21.59 U1.9
  Bottom 0.406: v73.66,22.86 72.39,21.59 70.48,21.59 69.85,22.23 52.07,22.23 49.53,24.77 U1.9
RA3  (via drill 0.6)
  Top 0.406: U6.11 72.39,10.79 76.2,10.79 76.2,14.61 v78.11,16.51 | U3.5 64.77,27.3 66.04,26.04 66.04,15.88 67.95,15.88 v67.95,13.97 | U5.11 44.45,14.61 45.72,15.88 45.72,19.05 40,19.05 40,19.69 38.1,19.69 38.1,22.23 39.37,23.5 U1.12
  Bottom 0.406: v78.11,16.51 74.93,16.51 74.93,19.69 74.3,20.32 69.22,20.32 68.58,20.96 50.8,20.96 50.16,21.59 45.09,21.59 45.09,23.5 40.64,23.5 U1.12 | v67.95,13.97 68.58,13.34 71.12,13.34 71.12,12.07 U6.11
RA4  (via drill 0.6)
  Top 0.406: U6.8 71.12,4.45 71.12,6.35 63.5,6.35 63.5,3.17 45.72,3.17 U5.8 43.18,3.17 40.64,3.17 40.64,6.35 35.56,11.43 35.56,27.3 36.83,28.57 U2.4 | v76.84,7.62 76.84,12.7 79.38,15.24 79.38,17.78 75.56,17.78 75.56,26.67 76.2,26.67 76.2,31.12 74.93,31.12 74.93,34.29 69.85,34.29 U3.14
  Bottom 0.406: U6.8 72.39,5.71 76.2,5.71 76.2,3.17 79.38,3.17 79.38,5.71 77.47,5.71 77.47,7.62 v76.84,7.62
RA5  (via drill 0.6)
  Top 0.406: v74.3,7.62 74.3,8.89 68.58,8.89 68.58,12.7 69.22,13.34 69.22,15.24 68.58,15.88 68.58,26.04 66.04,28.57 66.04,32.38 69.85,32.38 U3.7 | v41.91,32.38 44.45,32.38 U2.7
  Bottom 0.406: U5.7 43.18,4.45 43.18,5.71 52.7,5.71 52.7,3.17 66.04,3.17 66.04,5.71 69.85,5.71 | 69.85,5.71 U6.7 | 69.85,5.71 69.85,7.62 v74.3,7.62 | U3.7 69.85,32.38 67.31,32.38 66.67,31.75 52.7,31.75 52.7,30.48 48.89,30.48 48.89,32.38 v41.91,32.38
RA6  (via drill 0.6)
  Top 0.406: U6.6 67.31,2.54 40,2.54 39.37,3.17 U5.6 | v55.88,36.2 55.88,38.73 52.07,38.73 52.07,19.69 55.88,19.69 55.88,13.34 58.42,13.34 58.42,10.79 60.96,10.79 60.96,13.34 63.5,13.34 63.5,7.62 73.03,7.62 73.03,6.35 74.93,6.35 74.93,5.71 77.47,5.71 v77.47,4.45
  Bottom 0.406: U2.9 48.26,36.2 v55.88,36.2 73.66,36.2 U3.12 | v77.47,4.45 76.84,5.08 76.84,6.35 71.12,6.35 71.12,3.17 67.31,3.17 U6.6
RA7
  Top 0.406: U3.9 U6.10 | U2.12 40.64,37.46 40.64,31.12 43.18,31.12 43.18,23.5 41.27,23.5 41.27,19.69 48.26,19.69 48.26,15.88 46.99,14.61 U5.10
  Bottom 0.406: U6.10 73.66,13.34 71.76,13.34 71.76,14.61 69.85,14.61 69.85,15.24 66.67,15.24 66.67,13.34 52.7,13.34 51.43,12.07 U5.10
RG#  (1 unrouted)
  Top 0.406: U7.9 103.82,12.07 103.82,15.88 JP2.19
  Bottom 0.406: U9.8 101.6,55.24 83.82,55.24 83.82,59.05 66.67,59.05 66.04,59.69 50.8,59.69 50.16,60.32 JP1.20
RONLY  (via drill 0.6)  (1 unrouted)
  Top 0.406: JP2.22 107.95,12.07 107.95,6.98 96.52,6.98 95.25,5.71 U7.6 | U11.4 60.96,59.05 59.69,57.78 v59.69,52.7
  Bottom 0.406: v59.69,52.7 50.8,52.7 50.8,56.52 46.99,56.52 JP1.21
S$6
  Top 0.406: U9.1 86.36,51.43 87.63,52.7 87.63,58.42 88.9,59.69 U12.2
S$7  (via drill 0.6)
  other vias: 92.71,78.11
S$8  (via drill 0.6)
  other vias: 97.79,75.56
S$9  (via drill 0.6)
  other vias: 87.63,73.02
S$13  (via drill 0.6)
  other vias: 67.31,60.32
S$14  (via drill 0.6)
  other vias: 66.04,79.38
S$15  (via drill 0.6)
  other vias: 53.34,79.38
S$17  (via drill 0.6)
  other vias: 57.15,55.24
S$18  (via drill 0.6)
  other vias: 58.42,51.43
S$19  (via drill 0.6)
  other vias: 59.69,52.7
S$20  (via drill 0.6)
  other vias: 63.5,53.97
S$21  (via drill 0.6)
  other vias: 66.04,53.97
S$22  (via drill 0.6)
  other vias: 66.04,51.43
S$23  (via drill 0.6)
  other vias: 63.5,58.42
